| Teraspeed Modeling Services.
| http://www.teraspeed.com
[IBIS Ver]  3.2
[File Name] adc10d1000_292bga.ibs
[File Rev]  3.0
[Source]  Created by Teraspeed Consulting Group LLC
[Date]   07/30/2008
[Notes]   Quality Check of this IBIS model: Model Passes IBIS Check
   Model parses into ICX IS. Simulation done with Hyperlynx.
   1. MIN TYP MAX information is based on Temperature and
   Voltage characteristics only.
   2. Package data gained using TDA Systems Iconnect Software.
[Disclaimer]
|(C) Copyright National Semiconductor Corporation 2008
|   All rights reserved
|   National Semiconductor Corporation hereby grants
|the user of this IBIS model a non-exclusive, nontransferable
|license to use this IBIS model under the following terms.
|Before using this IBIS model, the user should read this
|license.  If the user does not accept these terms,  the
|IBIS model should be returned to National within 30 days.
|   The user is granted this license only to use the
|IBIS model and is not granted rights to sell, load, rent,
|lease or license the IBIS model in whole or in part, or in
|modified form to anyone other than user. User may modify
|the IBIS model to suit its specific applications but rights
|to derivative works and such modifications shall belong to
|National.
|   This IBIS model is provided on an "AS IS" basis and
|National makes absolutely no warranty with respect to the
|information contained herein.NATIONAL DISCLAIMS AND CUSTOMER
|WAIVES ALL WARRANTIES, EXPRESS OR IMPLIED, INCLUDING
|WARRANTIES OF MERCHANTABILITY OR FITNESS FOR A PARTICULAR
|PURPOSE. The entire risk as to quality and performance is
|with the Customer. ACCORDINGLY, IN NO EVENT SHALL THE
|COMPANY BE LIABLE FOR ANY DAMAGES, WHETHER IN CONTRACT OR
|TORT,INCLUDING ANY LOST PROFITS OR OTHER INCIDENTAL,
|CONSEQUENTIAL, EXEMPLARY, OR PUNITIVE DAMAGES ARISING OUT
|OF THE USE OR APPLICATION OF THE IBIS model provided in
|this package.Further, National reserves the right to make
|changes without notice to any product herein to improve
|reliability, function, or design. National does not convey
|any license under patent rights or any other intellectual
|property rights, including those of third parties.
|   National is not obligated to provide maintenance or support
|for the licensed IBIS model.
| Use: Teraspeed Consulting Group LLC ("Teraspeed") has
| licensed IBIS models to specific integrated circuit
| suppliers ("IC Vendors") for use and distribustion as
| follows: Each IC Vendor may use IBIS Models, and distribute
| them to IC Vendor's custumers to use solely for developing
| printed circute board designs. Users of this model may
| modify the IBIS model to suit its specific applications but
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[Copyright]
| This file is the legal property of National Semiconductor and
|	Teraspeed Copyright(c) 2008.
| All other rights are reserved.
[Component]   ADC10D1000_292BGA
[Manufacturer] National Semiconductor
[Package]
| variable   typ   min   max
R_pkg  9.111E-03   4.008E-03   1.234E-02
L_pkg  1.637E-09   1.074E-09   3.307E-09
C_pkg  8.281E-13   5.411E-13   1.666E-12
[Pin] signal_name  model_name  R_pin  L_pin C_pin
A1   GND   GND   1.000E-02 1.220E-09 6.210E-13
A2   V_A   POWER   1.000E-02 1.220E-09 6.210E-13
A3   SDO   out_tri   1.149E-02 3.080E-09 1.552E-12
A4   TPM   input   1.071E-02 2.871E-09 1.446E-12
A5   NDM   input   1.000E-02 2.680E-09 1.350E-12
A6   V_A   POWER   1.000E-02 1.220E-09 6.210E-13
A7   GND   GND   1.000E-02 1.220E-09 6.210E-13
A8   V_E   POWER   1.000E-02 1.220E-09 6.210E-13
A9   GND_E   GND   1.000E-02 1.220E-09 6.210E-13
A10   RSV0+   NC   1.000E-02 1.220E-09 6.210E-13
A11   V_DR   POWER   1.000E-02 1.220E-09 6.210E-13
A12   DId1+   lvds_hs   8.089E-03 2.168E-09 1.092E-12
A13   GND_DR   GND   1.000E-02 1.220E-09 6.210E-13
A14   DId4+   lvds_hs   8.836E-03 2.368E-09 1.193E-12
A15   V_DR   POWER   1.000E-02 1.220E-09 6.210E-13
A16   DId7+   lvds_hs   1.000E-02 2.680E-09 1.350E-12
A17   GND_DR   GND   1.000E-02 1.220E-09 6.210E-13
A18   DId9+   lvds_hs   1.149E-02 3.080E-09 1.552E-12
A19   DId9-   lvds_hs   1.234E-02 3.307E-09 1.666E-12
A20   GND_DR   GND   1.000E-02 1.220E-09 6.210E-13
B1   Vbg   term   1.234E-02 3.307E-09 1.666E-12
B2   GND   GND   1.000E-02 1.220E-09 6.210E-13
B3   ECEb   in_pu   1.050E-02 2.813E-09 1.417E-12
B4   SDI   input   9.660E-03 2.589E-09 1.304E-12
B5   CalRun   output   8.897E-03 2.384E-09 1.201E-12
B6   V_A   POWER   1.000E-02 1.220E-09 6.210E-13
B7   GND   GND   1.000E-02 1.220E-09 6.210E-13
B8   GND_E   GND   1.000E-02 1.220E-09 6.210E-13
B9   V_E   POWER   1.000E-02 1.220E-09 6.210E-13
B10   RSV0-   NC   1.000E-02 1.220E-09 6.210E-13
B11   DId0+   lvds_hs   6.598E-03 1.768E-09 8.907E-13
B12   DId1-   lvds_hs   6.812E-03 1.826E-09 9.197E-13
B13   DId3+   lvds_hs   7.161E-03 1.919E-09 9.668E-13
B14   DId4-   lvds_hs   7.634E-03 2.046E-09 1.031E-12
B15   DId6+   lvds_hs   8.217E-03 2.202E-09 1.109E-12
B16   DId7-   lvds_hs   8.897E-03 2.384E-09 1.201E-12
B17   DId8+   lvds_hs   9.660E-03 2.589E-09 1.304E-12
B18   RSV2+   NC   1.000E-02 1.220E-09 6.210E-13
B19   RSV3+   NC   1.000E-02 1.220E-09 6.210E-13
B20   RSV3-   NC   1.000E-02 1.220E-09 6.210E-13
C1   Rtrim+   term   1.149E-02 3.080E-09 1.552E-12
C2   Vcmo   term   1.050E-02 2.813E-09 1.417E-12
C3   Rext+   term   9.546E-03 2.558E-09 1.289E-12
C4   SCSb   input   8.653E-03 2.319E-09 1.168E-12
C5   SCLK   input   7.831E-03 2.099E-09 1.057E-12
C6   V_A   POWER   1.000E-02 1.220E-09 6.210E-13
C7   NC   POWER   1.000E-02 1.220E-09 6.210E-13
C8   V_E   POWER   1.000E-02 1.220E-09 6.210E-13
C9   GND_E   GND   1.000E-02 1.220E-09 6.210E-13
C10   RSV1+   NC   1.000E-02 1.220E-09 6.210E-13
C11   DId0-   lvds_hs   5.302E-03 1.421E-09 7.158E-13
C12   DId2+   lvds_hs   5.542E-03 1.485E-09 7.482E-13
C13   DId3-   lvds_hs   5.931E-03 1.589E-09 8.006E-13
C14   DId5+   lvds_hs   6.453E-03 1.729E-09 8.712E-13
C15   DId6-   lvds_hs   7.092E-03 1.901E-09 9.574E-13
C16   DId8-   lvds_hs   7.831E-03 2.099E-09 1.057E-12
C17   RSV2-   NC   1.000E-02 1.220E-09 6.210E-13
C18   V_DR   POWER   1.000E-02 1.220E-09 6.210E-13
C19   DI0+   lvds_hs   1.050E-02 2.813E-09 1.417E-12
C20   DI0-   lvds_hs   1.149E-02 3.080E-09 1.552E-12
D1   DNC   NC   1.000E-02 1.220E-09 6.210E-13
D2   Rtrim-   term   9.660E-03 2.589E-09 1.304E-12
D3   Rext-   term   8.653E-03 2.319E-09 1.168E-12
D4   GND   GND   1.000E-02 1.220E-09 6.210E-13
D5   GND   GND   1.000E-02 1.220E-09 6.210E-13
D6   CAL   input   6.007E-03 1.610E-09 8.109E-13
D7   DNC   term   5.302E-03 1.421E-09 7.158E-13
D8   V_A   POWER   1.000E-02 1.220E-09 6.210E-13
D9   V_A   POWER   1.000E-02 1.220E-09 6.210E-13
D10   RSV1-   NC   1.000E-02 1.220E-09 6.210E-13
D11   V_DR   POWER   1.000E-02 1.220E-09 6.210E-13
D12   DId2-   lvds_hs   4.281E-03 1.147E-09 5.779E-13
D13   GND_DR   GND   1.000E-02 1.220E-09 6.210E-13
D14   DId5-   lvds_hs   5.302E-03 1.421E-09 7.158E-13
D15   V_DR   POWER   1.000E-02 1.220E-09 6.210E-13
D16   GND_DR   GND   1.000E-02 1.220E-09 6.210E-13
D17   V_DR   POWER   1.000E-02 1.220E-09 6.210E-13
D18   DI1+   lvds_hs   8.653E-03 2.319E-09 1.168E-12
D19   DI2+   lvds_hs   9.660E-03 2.589E-09 1.304E-12
D20   DI2-   lvds_hs   1.071E-02 2.871E-09 1.446E-12
E1   V_A   POWER   1.000E-02 1.220E-09 6.210E-13
E2   Tdiode+   term   8.897E-03 2.384E-09 1.201E-12
E3   DNC   NC   1.000E-02 1.220E-09 6.210E-13
E4   GND   GND   1.000E-02 1.220E-09 6.210E-13
E17   GND_DR   GND   1.000E-02 1.220E-09 6.210E-13
E18   DI1-   lvds_hs   7.831E-03 2.099E-09 1.057E-12
E19   DI3+   lvds_hs   8.897E-03 2.384E-09 1.201E-12
E20   DI3-   lvds_hs   1.000E-02 2.680E-09 1.350E-12
F1   V_A   POWER   1.000E-02 1.220E-09 6.210E-13
F2   GND_TC   GND   1.000E-02 1.220E-09 6.210E-13
F3   Tdiode-   term   7.092E-03 1.901E-09 9.574E-13
F4   DNC   NC   1.000E-02 1.220E-09 6.210E-13
F17   GND_DR   GND   1.000E-02 1.220E-09 6.210E-13
F18   DI4+   lvds_hs   7.092E-03 1.901E-09 9.574E-13
F19   DI4-   lvds_hs   8.217E-03 2.202E-09 1.109E-12
F20   GND_DR   GND   1.000E-02 1.220E-09 6.210E-13
G1   V_TC   POWER   1.000E-02 1.220E-09 6.210E-13
G2   GND_TC   GND   1.000E-02 1.220E-09 6.210E-13
G3   V_TC   POWER   1.000E-02 1.220E-09 6.210E-13
G4   V_TC   POWER   1.000E-02 1.220E-09 6.210E-13
G17   DI5+   lvds_hs   5.302E-03 1.421E-09 7.158E-13
G18   DI5-   lvds_hs   6.453E-03 1.729E-09 8.712E-13
G19   DI6+   lvds_hs   7.634E-03 2.046E-09 1.031E-12
G20   DI6-   lvds_hs   8.836E-03 2.368E-09 1.193E-12
H1   VinI+   term   8.406E-03 2.253E-09 1.135E-12
H2   V_TC   POWER   1.000E-02 1.220E-09 6.210E-13
H3   GND_TC   GND   1.000E-02 1.220E-09 6.210E-13
H4   V_A   POWER   1.000E-02 1.220E-09 6.210E-13
H8   GND   GND   1.000E-02 1.220E-09 6.210E-13
H9   GND   GND   1.000E-02 1.220E-09 6.210E-13
H10   GND   GND   1.000E-02 1.220E-09 6.210E-13
H11   GND   GND   1.000E-02 1.220E-09 6.210E-13
H12   GND   GND   1.000E-02 1.220E-09 6.210E-13
H13   GND   GND   1.000E-02 1.220E-09 6.210E-13
H17   DI7+   lvds_hs   4.719E-03 1.265E-09 6.371E-13
H18   DI7-   lvds_hs   5.931E-03 1.589E-09 8.006E-13
H19   DI8+   lvds_hs   7.161E-03 1.919E-09 9.668E-13
H20   DI8-   lvds_hs   8.406E-03 2.253E-09 1.135E-12
J1   VinI-   term   8.089E-03 2.168E-09 1.092E-12
J2   GND_TC   GND   1.000E-02 1.220E-09 6.210E-13
J3   V_TC   POWER   1.000E-02 1.220E-09 6.210E-13
J4   VbiasI   term   4.281E-03 1.147E-09 5.779E-13
J8   GND   GND   1.000E-02 1.220E-09 6.210E-13
J9   GND   GND   1.000E-02 1.220E-09 6.210E-13
J10   GND   GND   1.000E-02 1.220E-09 6.210E-13
J11   GND   GND   1.000E-02 1.220E-09 6.210E-13
J12   GND   GND   1.000E-02 1.220E-09 6.210E-13
J13   GND   GND   1.000E-02 1.220E-09 6.210E-13
J17   V_DR   POWER   1.000E-02 1.220E-09 6.210E-13
J18   DI9+   lvds_hs   5.542E-03 1.485E-09 7.482E-13
J19   DI9-   lvds_hs   6.812E-03 1.826E-09 9.197E-13
J20   V_DR   POWER   1.000E-02 1.220E-09 6.210E-13
K1   GND   GND   1.000E-02 1.220E-09 6.210E-13
K2   VbiasI   term   6.598E-03 1.768E-09 8.907E-13
K3   V_TC   POWER   1.000E-02 1.220E-09 6.210E-13
K4   GND_TC   GND   1.000E-02 1.220E-09 6.210E-13
K8   GND   GND   1.000E-02 1.220E-09 6.210E-13
K9   GND   GND   1.000E-02 1.220E-09 6.210E-13
K10   GND   GND   1.000E-02 1.220E-09 6.210E-13
K11   GND   GND   1.000E-02 1.220E-09 6.210E-13
K12   GND   GND   1.000E-02 1.220E-09 6.210E-13
K13   GND   GND   1.000E-02 1.220E-09 6.210E-13
K17   ORI+   lvds_hs   4.008E-03 1.074E-09 5.411E-13
K18   ORI-   lvds_hs   5.302E-03 1.421E-09 7.158E-13
K19   DCLK_I+   lvds_hs   6.598E-03 1.768E-09 8.907E-13
K20   DCLK_I-   lvds_hs   7.896E-03 2.116E-09 1.066E-12
L1   GND   GND   1.000E-02 1.220E-09 6.210E-13
L2   VbiasQ   term   6.598E-03 1.768E-09 8.907E-13
L3   V_TC   POWER   1.000E-02 1.220E-09 6.210E-13
L4   GND_TC   GND   1.000E-02 1.220E-09 6.210E-13
L8   GND   GND   1.000E-02 1.220E-09 6.210E-13
L9   GND   GND   1.000E-02 1.220E-09 6.210E-13
L10   GND   GND   1.000E-02 1.220E-09 6.210E-13
L11   GND   GND   1.000E-02 1.220E-09 6.210E-13
L12   GND   GND   1.000E-02 1.220E-09 6.210E-13
L13   GND   GND   1.000E-02 1.220E-09 6.210E-13
L17   ORQ+   lvds_hs   4.008E-03 1.074E-09 5.411E-13
L18   ORQ-   lvds_hs   5.302E-03 1.421E-09 7.158E-13
L19   DCLK_Q+   lvds_hs   6.598E-03 1.768E-09 8.907E-13
L20   DCLK_Q-   lvds_hs   7.896E-03 2.116E-09 1.066E-12
M1   VinQ-   term   8.089E-03 2.168E-09 1.092E-12
M2   GND_TC   GND   1.000E-02 1.220E-09 6.210E-13
M3   V_TC   POWER   1.000E-02 1.220E-09 6.210E-13
M4   VbiasQ   term   4.281E-03 1.147E-09 5.779E-13
M8   GND   GND   1.000E-02 1.220E-09 6.210E-13
M9   GND   GND   1.000E-02 1.220E-09 6.210E-13
M10   GND   GND   1.000E-02 1.220E-09 6.210E-13
M11   GND   GND   1.000E-02 1.220E-09 6.210E-13
M12   GND   GND   1.000E-02 1.220E-09 6.210E-13
M13   GND   GND   1.000E-02 1.220E-09 6.210E-13
M17   GND_DR   GND   1.000E-02 1.220E-09 6.210E-13
M18   DQ9+   lvds_hs   5.542E-03 1.485E-09 7.482E-13
M19   DQ9-   lvds_hs   6.812E-03 1.826E-09 9.197E-13
M20   GND_DR   GND   1.000E-02 1.220E-09 6.210E-13
N1   VinQ+   term   8.406E-03 2.253E-09 1.135E-12
N2   V_TC   POWER   1.000E-02 1.220E-09 6.210E-13
N3   GND_TC   GND   1.000E-02 1.220E-09 6.210E-13
N4   V_A   POWER   1.000E-02 1.220E-09 6.210E-13
N8   GND   GND   1.000E-02 1.220E-09 6.210E-13
N9   GND   GND   1.000E-02 1.220E-09 6.210E-13
N10   GND   GND   1.000E-02 1.220E-09 6.210E-13
N11   GND   GND   1.000E-02 1.220E-09 6.210E-13
N12   GND   GND   1.000E-02 1.220E-09 6.210E-13
N13   GND   GND   1.000E-02 1.220E-09 6.210E-13
N17   DQ7+   lvds_hs   4.719E-03 1.265E-09 6.371E-13
N18   DQ7-   lvds_hs   5.931E-03 1.589E-09 8.006E-13
N19   DQ8+   lvds_hs   7.161E-03 1.919E-09 9.668E-13
N20   DQ8-   lvds_hs   8.406E-03 2.253E-09 1.135E-12
P1   V_TC   POWER   1.000E-02 1.220E-09 6.210E-13
P2   GND_TC   GND   1.000E-02 1.220E-09 6.210E-13
P3   V_TC   POWER   1.000E-02 1.220E-09 6.210E-13
P4   V_TC   POWER   1.000E-02 1.220E-09 6.210E-13
P17   DQ5+   lvds_hs   5.302E-03 1.421E-09 7.158E-13
P18   DQ5-   lvds_hs   6.453E-03 1.729E-09 8.712E-13
P19   DQ6+   lvds_hs   7.634E-03 2.046E-09 1.031E-12
P20   DQ6-   lvds_hs   8.836E-03 2.368E-09 1.193E-12
R1   V_A   POWER   1.000E-02 1.220E-09 6.210E-13
R2   GND_TC   GND   1.000E-02 1.220E-09 6.210E-13
R3   V_TC   POWER   1.000E-02 1.220E-09 6.210E-13
R4   V_TC   POWER   1.000E-02 1.220E-09 6.210E-13
R17   V_DR   POWER   1.000E-02 1.220E-09 6.210E-13
R18   DQ4+   lvds_hs   7.092E-03 1.901E-09 9.574E-13
R19   DQ4-   lvds_hs   8.217E-03 2.202E-09 1.109E-12
R20   V_DR   POWER   1.000E-02 1.220E-09 6.210E-13
T1   V_A   POWER   1.000E-02 1.220E-09 6.210E-13
T2   GND_TC   GND   1.000E-02 1.220E-09 6.210E-13
T3   GND_TC   GND   1.000E-02 1.220E-09 6.210E-13
T4   GND   GND   1.000E-02 1.220E-09 6.210E-13
T17   V_DR   POWER   1.000E-02 1.220E-09 6.210E-13
T18   DQ1-   lvds_hs   7.831E-03 2.099E-09 1.057E-12
T19   DQ3+   lvds_hs   8.897E-03 2.384E-09 1.201E-12
T20   DQ3-   lvds_hs   1.000E-02 2.680E-09 1.350E-12
U1   GND_TC   GND   1.000E-02 1.220E-09 6.210E-13
U2   CLK+   in_clk   9.660E-03 2.589E-09 1.304E-12
U3   PDI   in_pu   8.653E-03 2.319E-09 1.168E-12
U4   GND   GND   1.000E-02 1.220E-09 6.210E-13
U5   GND   GND   1.000E-02 1.220E-09 6.210E-13
U6   RCOut_1-  lvds_ls   6.007E-03 1.610E-09 8.109E-13
U7   DNC   term   5.302E-03 1.421E-09 7.158E-13
U8   V_A   POWER   1.000E-02 1.220E-09 6.210E-13
U9   V_A   POWER   1.000E-02 1.220E-09 6.210E-13
U10   RSV7-   NC   1.000E-02 1.220E-09 6.210E-13
U11   V_DR   POWER   1.000E-02 1.220E-09 6.210E-13
U12   DQd2-   lvds_hs   4.281E-03 1.147E-09 5.779E-13
U13   GND_DR   GND   1.000E-02 1.220E-09 6.210E-13
U14   DQd5-   lvds_hs   5.302E-03 1.421E-09 7.158E-13
U15   V_DR   POWER   1.000E-02 1.220E-09 6.210E-13
U16   V_DR   POWER   1.000E-02 1.220E-09 6.210E-13
U17   GND_DR   GND   1.000E-02 1.220E-09 6.210E-13
U18   DQ1+   lvds_hs   8.653E-03 2.319E-09 1.168E-12
U19   DQ2+   lvds_hs   9.660E-03 2.589E-09 1.304E-12
U20   DQ2-   lvds_hs   1.071E-02 2.871E-09 1.446E-12
V1   CLK-   in_clk   1.149E-02 3.080E-09 1.552E-12
V2   DCLK_RST+ in_clk   1.050E-02 2.813E-09 1.417E-12
V3   PDQ   in_pu   9.546E-03 2.558E-09 1.289E-12
V4   CalDly   input   8.653E-03 2.319E-09 1.168E-12
V5   DES   input   7.831E-03 2.099E-09 1.057E-12
V6   RCOut_2+  lvds_ls   7.092E-03 1.901E-09 9.574E-13
V7   RCOut_2-  lvds_ls   6.453E-03 1.729E-09 8.712E-13
V8   V_E   POWER   1.000E-02 1.220E-09 6.210E-13
V9   GND_E   GND   1.000E-02 1.220E-09 6.210E-13
V10   RSV7+   NC   1.000E-02 1.220E-09 6.210E-13
V11   DQd0-   lvds_hs   5.302E-03 1.421E-09 7.158E-13
V12   DQd2+   lvds_hs   5.542E-03 1.485E-09 7.482E-13
V13   DQd3-   lvds_hs   5.931E-03 1.589E-09 8.006E-13
V14   DQd5+   lvds_hs   6.453E-03 1.729E-09 8.712E-13
V15   DQd6-   lvds_hs   7.092E-03 1.901E-09 9.574E-13
V16   DQd8-   lvds_hs   7.831E-03 2.099E-09 1.057E-12
V17   RSV4-   NC   1.000E-02 1.220E-09 6.210E-13
V18   GND_DR   GND   1.000E-02 1.220E-09 6.210E-13
V19   DQ0+   lvds_hs   1.050E-02 2.813E-09 1.417E-12
V20   DQ0-   lvds_hs   1.149E-02 3.080E-09 1.552E-12
W1   DCLK_RST- in_clk   1.234E-02 3.307E-09 1.666E-12
W2   GND   GND   1.000E-02 1.220E-09 6.210E-13
W3   DNC   NC   1.000E-02 1.220E-09 6.210E-13
W4   DDRPh   input   9.660E-03 2.589E-09 1.304E-12
W5   RCLK-   in_clk   8.897E-03 2.384E-09 1.201E-12
W6   V_A   POWER   1.000E-02 1.220E-09 6.210E-13
W7   GND   GND   1.000E-02 1.220E-09 6.210E-13
W8   GND_E   GND   1.000E-02 1.220E-09 6.210E-13
W9   V_E   POWER   1.000E-02 1.220E-09 6.210E-13
W10   RSV6-   NC   1.000E-02 1.220E-09 6.210E-13
W11   DQd0+   lvds_hs   6.598E-03 1.768E-09 8.907E-13
W12   DQd1-   lvds_hs   6.812E-03 1.826E-09 9.197E-13
W13   DQd3+   lvds_hs   7.161E-03 1.919E-09 9.668E-13
W14   DQd4-   lvds_hs   7.634E-03 2.046E-09 1.031E-12
W15   DQd6+   lvds_hs   8.217E-03 2.202E-09 1.109E-12
W16   DQd7-   lvds_hs   8.897E-03 2.384E-09 1.201E-12
W17   DQd8+   lvds_hs   9.660E-03 2.589E-09 1.304E-12
W18   RSV4+   NC   1.000E-02 1.220E-09 6.210E-13
W19   RSV5+   NC   1.000E-02 1.220E-09 6.210E-13
W20   RSV5-   NC   1.000E-02 1.220E-09 6.210E-13
Y1   GND   GND   1.000E-02 1.220E-09 6.210E-13
Y2   V_A   POWER   1.000E-02 1.220E-09 6.210E-13
Y3   FSR   input   1.149E-02 3.080E-09 1.552E-12
Y4   RCLK+   in_clk   1.071E-02 2.871E-09 1.446E-12
Y5   RCOut_1+  lvds_ls   1.000E-02 2.680E-09 1.350E-12
Y6   V_A   POWER   1.000E-02 1.220E-09 6.210E-13
Y7   GND   GND   1.000E-02 1.220E-09 6.210E-13
Y8   V_E   POWER   1.000E-02 1.220E-09 6.210E-13
Y9   GND_E   GND   1.000E-02 1.220E-09 6.210E-13
Y10   RSV6+   NC   1.000E-02 1.220E-09 6.210E-13
Y11   V_DR   POWER   1.000E-02 1.220E-09 6.210E-13
Y12   DQd1+   lvds_hs   8.089E-03 2.168E-09 1.092E-12
Y13   GND_DR   GND   1.000E-02 1.220E-09 6.210E-13
Y14   DQd4+   lvds_hs   8.836E-03 2.368E-09 1.193E-12
Y15   V_DR   POWER   1.000E-02 1.220E-09 6.210E-13
Y16   DQd7+   lvds_hs   1.000E-02 2.680E-09 1.350E-12
Y17   GND_DR   GND   1.000E-02 1.220E-09 6.210E-13
Y18   DQd9+   lvds_hs   1.149E-02 3.080E-09 1.552E-12
Y19   DQd9-   lvds_hs   1.234E-02 3.307E-09 1.666E-12
Y20   GND_DR   GND   1.000E-02 1.220E-09 6.210E-13
[Diff Pin] inv_pin vdiff tdelay_typ tdelay_min tdelay_max
U2   V1   200mV NA   NA   NA
V2   W1   200mV NA   NA   NA
Y4   W5   200mV NA   NA   NA
A12   B12   NA   NA   NA   NA
A14   B14   NA   NA   NA   NA
A16   B16   NA   NA   NA   NA
A18   A19   NA   NA   NA   NA
B11   C11   NA   NA   NA   NA
B13   C13   NA   NA   NA   NA
B15   C15   NA   NA   NA   NA
B17   C16   NA   NA   NA   NA
C1   D2   NA   NA   NA   NA
C12   D12   NA   NA   NA   NA
C14   D14   NA   NA   NA   NA
C19   C20   NA   NA   NA   NA
C3   D3   NA   NA   NA   NA
D18   E18   NA   NA   NA   NA
D19   D20   NA   NA   NA   NA
E19   E20   NA   NA   NA   NA
E2   F3   NA   NA   NA   NA
F18   F19   NA   NA   NA   NA
G17   G18   NA   NA   NA   NA
G19   G20   NA   NA   NA   NA
H1   J1   NA   NA   NA   NA
H17   H18   NA   NA   NA   NA
H19   H20   NA   NA   NA   NA
J18   J19   NA   NA   NA   NA
K17   K18   NA   NA   NA   NA
K19   K20   NA   NA   NA   NA
L17   L18   NA   NA   NA   NA
L19   L20   NA   NA   NA   NA
M18   M19   NA   NA   NA   NA
N1   M1   NA   NA   NA   NA
N17   N18   NA   NA   NA   NA
N19   N20   NA   NA   NA   NA
P17   P18   NA   NA   NA   NA
P19   P20   NA   NA   NA   NA
R18   R19   NA   NA   NA   NA
T19   T20   NA   NA   NA   NA
U18   T18   NA   NA   NA   NA
U19   U20   NA   NA   NA   NA
V12   U12   NA   NA   NA   NA
V14   U14   NA   NA   NA   NA
V19   V20   NA   NA   NA   NA
V6   V7   NA   NA   NA   NA
W11   V11   NA   NA   NA   NA
W13   V13   NA   NA   NA   NA
W15   V15   NA   NA   NA   NA
W17   V16   NA   NA   NA   NA
Y12   W12   NA   NA   NA   NA
Y14   W14   NA   NA   NA   NA
Y16   W16   NA   NA   NA   NA
Y18   Y19   NA   NA   NA   NA
Y5   U6   NA   NA   NA   NA
[Series Pin Mapping] pin_2 model_name function_table_group
H1   J1   100_ohm
N1   M1   100_ohm
U2   V1   100_ohm
V2   W1   100_ohm
Y4   W5   100_ohm
C3   D3   3300_ohm
C1   D2   3300_ohm
[Model Selector]  lvds_hs
lvds_lo_vbgf   output voltage=lo, vbg=floating
lvds_hi_vbgf   output voltage=hi, vbg=floating
lvds_lo_vbg1   output voltage=lo, vbg=hi
lvds_hi_vbg1   output voltage=hi, vbg=hi
[Model]   100_ohm
Model_type   Series
C_comp   0  0  0
[Temperature Range]   25   85   -40
|   typ   min   max
[Voltage Range]  1.9V 1.8V 2.0V
[R series]   100   94   106
[Model]   3300_ohm
Model_type   Series
C_comp   0  0  0
[Temperature Range]   25   85   -40
|   typ   min   max
[Voltage Range]  1.9V   1.8V   2.0V
[R series]   3300   3300   3300
[Model] term
Model_type Terminator
C_comp   0  0  0
| variable   typ   min   max
[Voltage Range]   1.900E+00   1.800E+00   2.000E+00
[POWER Clamp Reference]  1.900E+00   1.800E+00   2.000E+00
[GND Clamp Reference]   0.00000V   0.00000V   0.00000V
[Temperature Range]   25   85   -40
| Models and submodels in the file (13): in_clk (Input), in_pu (Input), input (Input), lvds_hi_vbg1 (Output), lvds_hi_vbgf (Output), lvds_lo_vbg1 (Output), lvds_lo_vbgf (Output), lvds_ls (Output), out_tri (3-state), output (Output), 100_ohm (Series), 3300_ohm (Series), term (Terminator)
